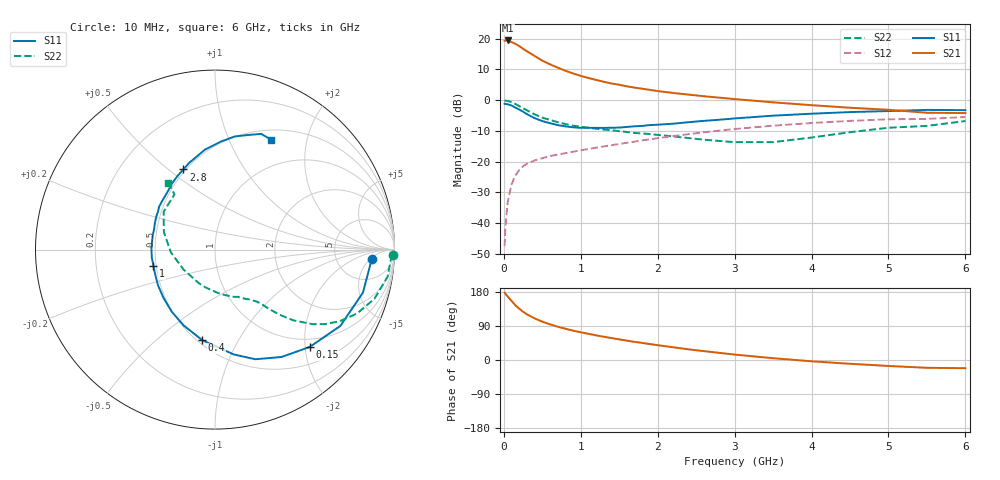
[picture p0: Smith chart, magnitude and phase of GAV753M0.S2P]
! Infineon Technologies  Discrete & RF Semiconductors
! BF775
! Si NPN RF Bipolar Junction Transistor in SOT23
! VCE = 0.75 V  IC = 3 mA
! Common Emitter S-Parameters:  May  1996
# GHz  S  MA  R  50
!  f  S11  S21  S12  S22
! GHz  MAG  ANG  MAG  ANG  MAG  ANG  MAG  ANG
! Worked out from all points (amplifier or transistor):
!   36 points, 10 MHz to 6 GHz, reference 50 ohm
!   highest |S21| = 19.4 dB at 50 MHz (marker M1)
!   |S21| within 3 dB of that: start of sweep to 267.6 MHz
!   unconditionally stable (mu >= 1): 873.5 MHz to end of sweep
!   at 250 MHz: K = 0.38, MSG = 19.1 dB, |S12| = -21.5 dB
!   at 1.4 GHz: K = 1.19, MAG = 7.4 dB, |S12| = -14.7 dB
!   at 6 GHz: K = 1.07, MAG = -0.9 dB, |S12| = -5.5 dB
!   S11 on the Smith chart (normalised r, x): 10 MHz: 12, -6; 150 MHz: 0.83, -2.10; 400 MHz: 0.53, -0.72; 1 GHz: 0.48, -0.10; 2.8 GHz: 0.49, +0.56; 6 GHz: 0.62, +1.44
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0.01  0.8745 -3.4  9.292 177.8  0.0042 89.3  0.9916 -1.7
0.02  0.8671 -6.5  9.348 174.8  0.0086 87.4  0.9808 -3.5
0.05  0.8584 -16.2  9.376 167.5  0.0219 80.8  0.973 -9.0
0.1  0.8178 -31.3  8.825 156.0  0.0426 72.7  0.9292 -17.2
0.15  0.7567 -45.8  8.274 144.3  0.0596 65.0  0.8671 -24.3
0.2  0.7039 -58.2  7.603 135.4  0.0728 59.6  0.8011 -29.9
0.25  0.651 -69.8  6.853 127.4  0.084 55.1  0.7403 -34.1
0.3  0.5926 -80.0  6.258 120.5  0.0924 51.8  0.6839 -37.4
0.4  0.5095 -98.0  5.247 109.9  0.1045 47.3  0.5878 -42.1
0.5  0.4571 -112.5  4.396 101.2  0.1137 45.1  0.5203 -44.8
0.6  0.4214 -125.0  3.832 94.1  0.1229 43.6  0.4762 -46.5
0.7  0.3929 -137.1  3.388 87.8  0.13 43.2  0.4387 -48.0
0.8  0.3746 -147.8  3.012 82.5  0.1374 43.1  0.4083 -49.1
1  0.3548 -165.0  2.487 73.2  0.1525 43.5  0.3691 -51.4
1.1  0.3549 -172.8  2.297 69.0  0.1606 43.4  0.356 -53.1
1.6  0.3669 155.7  1.679 51.0  0.2025 43.5  0.3033 -62.1
2.2  0.4135 130.4  1.31 33.6  0.2601 41.0  0.2569 -78.7
2.8  0.48 111.6  1.099 18.9  0.3195 35.9  0.2168 -104.4
3.5  0.5595 95.8  0.922 4.7  0.3842 27.7  0.2075 -147.5
4.5  0.64 80.1  0.753 -10.0  0.4603 14.9  0.301 161.1
5.5  0.6942 68.2  0.624 -20.6  0.4945 1.2  0.3813 126.3
6  0.6878 63.1  0.616 -21.6  0.5316 -2.6  0.4568 125.1
